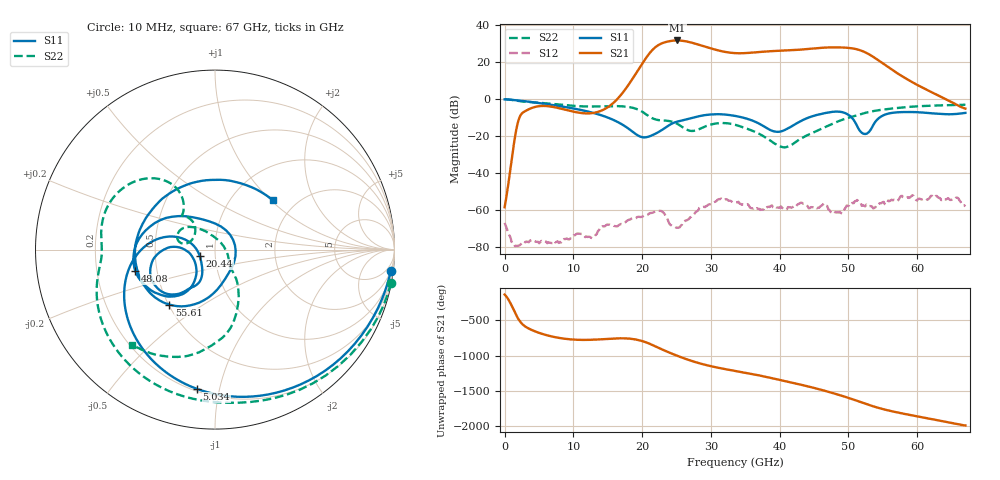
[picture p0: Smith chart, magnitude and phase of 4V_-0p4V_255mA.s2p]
! MARKI MICROWAVE INC.
! Date:  10/23/18
! Model Number:  AMM-6702CH
! Description:  2-port Small Signal S-parameter data for AMM-6702CH
! Frequency Range:  10 MHz to 67 GHz
! Port Configuration:  PORT 1: Input
!  PORT 2: Output
! Bias Condition: Vd = +4V, Vg = -0.4V
! AMM-6702CH s2p files are only valid for small signal conditions (below -5 dBm input power)
!S2P File: Measurements: Mag<S11> Ang<S11>, Mag<S21> Ang<S21>, Mag<S12> Ang<S12>, Mag<S22> Ang<S22>!row 1
# Hz S  dB  R 50
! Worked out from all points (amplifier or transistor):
!   401 points, 10 MHz to 67 GHz, reference 50 ohm
!   highest |S21| = 31.8 dB at 25.13 GHz (marker M1)
!   |S21| within 3 dB of that: 22.16 GHz to 28.84 GHz (6.673 GHz wide, 26.2 % of centre)
!   unconditionally stable (mu >= 1): start of sweep to end of sweep
!   at 11.06 GHz: K = 2292.57, MAG = -3.9 dB, |S12| = -73.0 dB
!   at 33.51 GHz: K = 14.86, MAG = 25.7 dB, |S12| = -55.9 dB
!   at 67 GHz: K = 297.70, MAG = -1.3 dB, |S12| = -58.1 dB
!   S11 on the Smith chart (normalised r, x): 10 MHz: 2, -17; 5.034 GHz: 0.21, -0.86; 20.44 GHz: 0.84, -0.06; 48.08 GHz: 0.38, -0.11; 55.61 GHz: 0.51, -0.37; 67 GHz: 1.53, +1.03
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1e7  -0.11 -6.8  -58.53 -136.0  -66.98 26.3  -0.02 -10.8
5.03425e9  -2.13 -97.4  -3.81 42.2  -78.04 -100.6  -1.95 -126.7
1.123082e10  -5.96 -165.3  -7.55 -57.0  -72.98 153.1  -3.90 -174.5
1.80973e10  -16.20 162.9  8.17 -38.8  -65.26 154.9  -4.30 144.6
2.044195e10  -20.70 -157.1  21.62 -87.2  -62.97 126.6  -7.87 122.1
2.161428e10  -19.31 -133.8  27.06 -134.0  -61.37 119.3  -10.55 125.9
2.245165e10  -17.69 -123.0  29.45 -172.0  -60.47 101.7  -11.40 132.0
2.362398e10  -14.87 -115.5  31.10 137.4  -64.34 56.4  -11.70 133.7
2.513125e10  -12.15 -121.5  31.77 77.9  -69.62 97.0  -13.43 128.8
2.6806e10  -10.62 -126.7  30.94 18.4  -64.92 125.7  -16.99 142.6
2.898318e10  -8.74 -137.9  28.60 -44.3  -58.29 121.6  -15.10 169.5
3.3505e10  -9.07 -170.2  24.91 -134.3  -55.90 43.5  -13.86 141.9
3.702198e10  -13.28 176.0  25.50 161.2  -59.40 41.1  -18.79 117.3
4.0204e10  -17.47 -144.8  26.26 93.4  -58.12 16.9  -25.76 56.6
4.238118e10  -13.29 -122.8  26.65 45.5  -58.00 41.6  -23.09 -16.0
4.472582e10  -9.30 -130.6  27.37 -8.6  -58.52 -138.7  -18.37 -46.7
4.807532e10  -6.75 -165.0  28.04 -98.3  -61.27 173.3  -12.67 -57.2
5.02525e10  -9.19 151.8  27.64 -164.5  -56.51 153.5  -9.81 -66.5
5.22622e10  -18.82 28.6  25.65 127.6  -57.77 -149.3  -7.65 -75.6
5.56117e10  -8.00 -129.6  17.75 30.4  -56.60 90.1  -5.38 -92.6
5.594665e10  -7.69 -134.7  16.90 22.8  -55.25 141.4  -5.23 -94.1
6.7e10  -7.46 40.8  -5.13 174.1  -58.07 59.5  -3.03 -130.8
